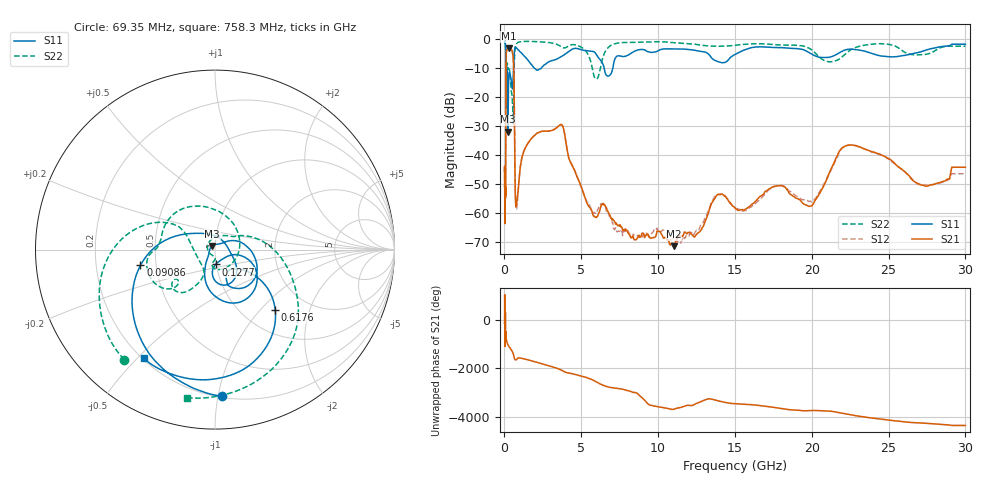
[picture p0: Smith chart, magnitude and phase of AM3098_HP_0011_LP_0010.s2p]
! Date/Time: Thu, Feb 28, 2019 8:33 AM
! Network Analyzer: Agilent Technologies E8364B Rev: A.07.50.67
! Sweep from 0.010 to 30.000 GHz, 1601 Points, Sweep Type: LOG
! Power Supply: 5.022 V, 0.002 A
# Hz S DB R 50
!freq MagS11 AngS11 MagS21 AngS21 MagS12 AngS12 MagS22 AngS22
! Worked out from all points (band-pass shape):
!   1601 points, 10 MHz to 30 GHz, reference 50 ohm
!   highest |S21| = -3.03 dB at 266.5 MHz (marker M1); lowest = -71.5 dB at 11.03 GHz (marker M2)
!   |S21| within 3 dB of the highest: 107.7 MHz to 562.8 MHz (455.1 MHz wide, 136 % of centre)
!   lowest |S11| = -31.9 dB at 228.2 MHz (marker M3), VSWR 1.05, Z = 48.4 + j1.96 ohm
!   |S11| at or under -10 dB: 175.7 MHz to 587.8 MHz (412.1 MHz wide, 108 % of centre); 1.967 GHz to 2.381 GHz (413.7 MHz wide, 19 % of centre); 6.494 GHz to 7.05 GHz (555.8 MHz wide, 8.21 % of centre)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
!   |S22| runs from -29.1 to -0.5 dB; largest |S21 - S12| = 0.011
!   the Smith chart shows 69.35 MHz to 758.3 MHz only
!   S11 on the Smith chart (normalised r, x): 69.35 MHz: 0.21, -1.03; 90.86 MHz: 0.41, -0.09; 127.7 MHz: 0.99, -0.17; 617.6 MHz: 1.40, -1.21; 758.3 MHz: 0.20, -0.52
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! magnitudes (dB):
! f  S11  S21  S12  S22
! 10 MHz  -0.3  -45.6  -44.1  -0.5
! 38.04 MHz  -0.5  -58.1  -59.2  -0.8
! 69.35 MHz  -1.7  -51.8  -54.8  -2.0
! 77.03 MHz  -2.4  -52.5  -48.8  -2.6
! 90.86 MHz  -7.4  -20.8  -20.8  -8.7
! 127.7 MHz  -21.6  -4.2  -4.2  -11.0
! 144.7 MHz  -14.3  -3.6  -3.6  -10.4
! 187.7 MHz  -11.6  -3.4  -3.5  -8.3
! 228.2 MHz  -31.9  -3.1  -3.1  -9.8
! 266.5 MHz  -15.0  -3.0  -3.0  -10.3
! 550.5 MHz  -14.9  -5.4  -5.4  -25.2
! 617.6 MHz  -6.5  -13.3  -13.3  -13.2
! 699.9 MHz  -2.7  -52.4  -51.6  -2.5
! 758.3 MHz  -2.8  -57.3  -57.2  -1.5
! 2.084 GHz  -10.5  -32.5  -32.6  -0.7
! 3.723 GHz  -5.8  -29.5  -29.5  -2.6
! 5.989 GHz  -5.3  -61.6  -59.7  -13.7
! 7.926 GHz  -5.7  -66.1  -65.7  -1.0
! 11.03 GHz  -3.3  -71.5  -68.9  -1.1
! 19.9 GHz  -4.8  -57.7  -55.9  -3.3
! 22.67 GHz  -3.4  -36.5  -36.6  -3.2
! 30 GHz  -1.6  -44.2  -46.4  -2.3
